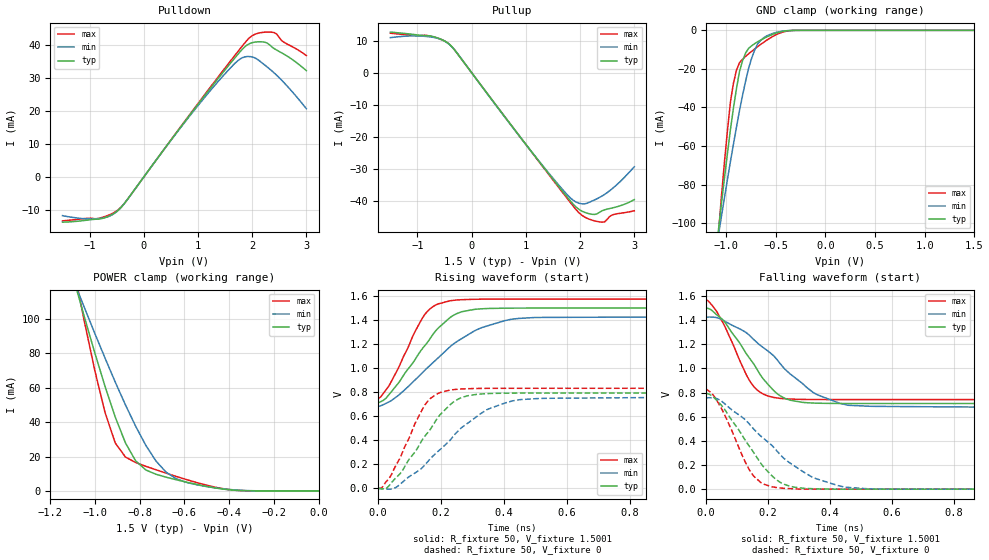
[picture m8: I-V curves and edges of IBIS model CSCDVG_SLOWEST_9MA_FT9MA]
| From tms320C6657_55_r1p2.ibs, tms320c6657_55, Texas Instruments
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|   Model Cell CSCDVG_SLOWEST_9MA_FT9MA
|SLOWEST_9MA
[Model]   CSCDVG_SLOWEST_9MA_FT9MA
Model_type   I/O
Polarity   Non-Inverting
Enable   Active-Low
Cref =  4.0000pF
Rref =  100.0000M
Vref =  0V
Vmeas =  0.75
C_comp   1.5249p   1.4275p   1.6205p
|[mode_tieoffpin] SR1=1  SR0=1 I0=1 I1=0 I2=1
[Model Spec]
Vinl   0.6125   0.6125   0.6125
Vinh   0.9625   0.9625   0.9625
D_overshoot_high 1.95 1.95 1.95
D_overshoot_low -0.3 -0.3 -0.3
D_overshoot_time 1E-9 1E-9 1E-9
S_overshoot_high 1.575 1.575 1.575
S_overshoot_low 0 0 0
[Receiver Thresholds]
Reference_supply Pullup_ref
Threshold_sensitivity= 0.5
Tslew_ac= 5nS
Vinh_ac= +175mV
Vinh_dc= +100mV
Vinl_ac= -175mV
Vinl_dc= -100mV
Vth = 0.75
Vth_max= 0.79
Vth_min= 0.71
[Pullup Reference] 1.5001   1.425   1.575
[Add Submodel]
|Submodel_name Mode
CSCDVG_FT_TH_9MA Non-Driving
[Temperature Range]   25   105   -40
[Voltage Range]   1.5   1.425   1.575
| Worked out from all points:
|   slope of the pulldown table from 0 to 0.225 V, typ, clamps not added: 44.4 ohm
|   slope of the pullup table from 0 to 0.225 V, typ, clamps not added: 44.4 ohm
|   GND clamp passes 1 mA (typ) near -0.47 V on its own axis
|   POWER clamp passes 1 mA (typ) near -0.42 V on its own axis
|   rising waveform, R_fixture 50, V_fixture 1.5001: 20-80 % time 133ps typ, 197ps min, 93.2ps max; typ from 0.71 V to 1.5 V
|   rising waveform, R_fixture 50, V_fixture 0: 20-80 % time 126ps typ, 187ps min, 90.7ps max; typ from 0 V to 0.793 V
|   falling waveform, R_fixture 50, V_fixture 1.5001: 20-80 % time 128ps typ, 194ps min, 90.3ps max; typ from 1.5 V to 0.709 V
|   falling waveform, R_fixture 50, V_fixture 0: 20-80 % time 128ps typ, 198ps min, 88.4ps max; typ from 0.793 V to 0 V
[POWER_clamp]
|   voltage   I(typ)   I(min)   I(max)
-1.5V     321.7mA    260.6mA    415.9mA
-1.076V   114.2mA    115.8mA    116.9mA
-1.061V   107.2mA    110.9mA    107.1mA
-954.6mV  60.59mA    77.06mA    45.35mA
-909.2mV  42.85mA    63.21mA    27.81mA
-863.7mV  27.9mA     49.99mA    19.69mA
-818.2mV  17.49mA    37.63mA    16.52mA
-772.8mV  12.19mA    26.53mA    14.33mA
-681.9mV  7.985mA    10.89mA    10.33mA
-590.9mV  5.094mA    4.955mA    6.6mA
-363.7mV  298.5uA    465.2uA    297.6uA
0V        1.518nA    24.08nA    367.8pA
[Pulldown]
|   voltage   I(typ)   I(min)   I(max)
-1.5V     -13.72mA   -11.73mA   -13.31mA
-863.7mV  -12.8mA    -12.65mA   -12.66mA
-500mV    -10.46mA   -10.55mA   -10.29mA
-318.2mV  -7.172mA   -7.186mA   -7.182mA
1.046V    23.05mA    22.61mA    23.31mA
1.591V    34.39mA    33mA       35.06mA
1.818V    38.82mA    36.24mA    39.81mA
1.955V    40.55mA    36.61mA    42.37mA
2.091V    41.08mA    35.83mA    43.61mA
2.273V    40.74mA    33.5mA     44.04mA
2.364V    39.55mA    32.26mA    43.99mA
3V        32.34mA    20.77mA    36.92mA
[Pullup]
|   voltage   I(typ)   I(min)   I(max)
-1.5V     12.66mA    10.94mA    12.31mA
-818.2mV  11.55mA    11.26mA    11.58mA
-590.9mV  10.61mA    10.52mA    10.54mA
-409.1mV  8.836mA    8.777mA    8.84mA
1.227V    -27.25mA   -27.19mA   -27.38mA
1.727V    -37.96mA   -37.32mA   -38.38mA
1.909V    -41.55mA   -40.1mA    -42.29mA
2.046V    -43.18mA   -40.84mA   -44.51mA
2.227V    -44.08mA   -39.9mA    -45.94mA
2.409V    -42.96mA   -38.35mA   -46.53mA
2.591V    -42.11mA   -36.14mA   -44.31mA
3V        -39.5mA    -29.28mA   -42.98mA
[GND_clamp]
|   voltage   I(typ)   I(min)   I(max)
-1.5V     -310.1mA   -250.5mA   -402.5mA
-1.076V   -103.6mA   -106.2mA   -105.2mA
-1.046V   -89.81mA   -96.36mA   -86.02mA
-954.6mV  -51.22mA   -67.87mA   -36.88mA
-924.3mV  -40.08mA   -58.86mA   -27.29mA
-863.7mV  -21.24mA   -41.56mA   -16.73mA
-833.4mV  -15.8mA    -33.75mA   -15.03mA
-772.8mV  -9.345mA   -19.75mA   -12.19mA
-712.2mV  -6.928mA   -10.35mA   -9.704mA
-621.3mV  -4.261mA   -3.896mA   -6.225mA
-409.1mV  -337.1uA   -289.1uA   -618.9uA
1.5V      1.518nA    257.2nA    299pA
[Ramp]
| variable   typ   min   max
dV/dt_f   0.632912/0.18543928n   0.59944/0.30124073n   0.666584/0.13417172n
dV/dt_r 0.63885392/0.18548444n 0.61071216/0.28637454n 0.66808936/0.13313997n
R_load = 50
[Rising Waveform]
R_fixture = 50
V_fixture = 1.5001
V_fixture_min = 1.425
V_fixture_max = 1.575
|   time   V(typ)   V(min)   V(max)
0s        709.9mV    677.9mV    742.7mV
35.96ps   785.4mV    721.7mV    860.4mV
115.9ps   1.066V     898.8mV    1.298V
145.6ps   1.179V     975.8mV    1.437V
180.9ps   1.304V     1.062V     1.522V
228.5ps   1.421V     1.178V     1.561V
266ps     1.47V      1.247V     1.57V
325.2ps   1.493V     1.333V     1.574V
445.9ps   1.5V       1.414V     1.575V
1.282ns   1.5V       1.425V     1.575V
[Rising Waveform]
R_fixture = 50
V_fixture = 0
V_fixture_min = 0
V_fixture_max = 0
|   time   V(typ)   V(min)   V(max)
0s        0V         0V         0V
25.81ps   0V         -5.884mV   56.92mV
68.17ps   117.3mV    30.35mV    245.7mV
116.7ps   301.5mV    127.2mV    536.8mV
153.6ps   451.1mV    210.1mV    711.8mV
226.6ps   689.9mV    394.2mV    816.8mV
265.7ps   755.6mV    505.6mV    827.2mV
345ps     788.1mV    653.4mV    831.9mV
450.6ps   792.5mV    738.1mV    832.6mV
1.29ns    793mV      756.2mV    832.8mV
[Falling Waveform]
R_fixture = 50
V_fixture = 1.5001
V_fixture_min = 1.425
V_fixture_max = 1.575
|   time   V(typ)   V(min)   V(max)
0s        1.499V     1.424V     1.575V
32.81ps   1.447V     1.422V     1.478V
55.23ps   1.399V     1.399V     1.374V
138.4ps   1.091V     1.278V     907.3mV
168.2ps   976.6mV    1.205V     814.6mV
201.1ps   864.5mV    1.142V     770.7mV
253.9ps   753mV      995.5mV    748.6mV
346.2ps   713.3mV    800.4mV    742.6mV
458.8ps   709.6mV    695mV      742mV
1.282ns   709.3mV    676.9mV    741.9mV
[Falling Waveform]
R_fixture = 50
V_fixture = 0
V_fixture_min = 0
V_fixture_max = 0
|   time   V(typ)   V(min)   V(max)
0s        792.6mV    755.6mV    831.9mV
26.46ps   755.7mV    754.5mV    768.3mV
52.33ps   685.8mV    724.3mV    654.9mV
148.1ps   324.5mV    514.2mV    126.7mV
175.3ps   219.5mV    442.6mV    58.45mV
211.3ps   114.7mV    365.5mV    20.8mV
262.1ps   31.27mV    233.1mV    5.334mV
342ps     3.945mV    100.9mV    0V
452.3ps   0V         15.76mV    0V
1.29ns    0V         0V         0V
